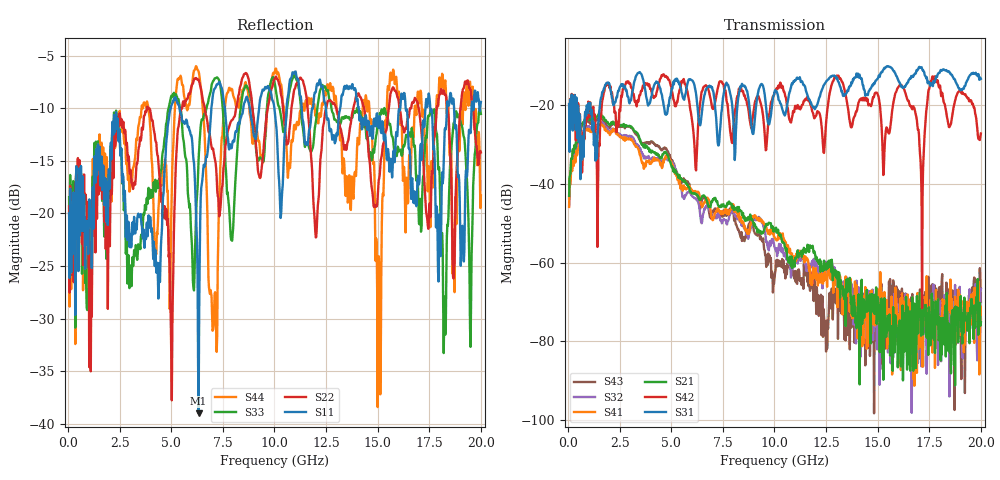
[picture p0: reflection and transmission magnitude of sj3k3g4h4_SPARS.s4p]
! FILE: E:\users\goganessyan\GBX_Backplane\FR408_backplane\1m_INBOUND_FEXT\sj3k3g4h4_SPARS.s4p
# MHZ S RI R 50.00
! FREQ  S11  S12  S13  S14
!  S21  S22  S23  S24
!  S31  S32  S33  S34
!  S41  S42  S43  S44
!  REAL  IMAG  REAL  IMAG  REAL  IMAG  REAL  IMAG
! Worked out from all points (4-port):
!   799 points, 50 MHz to 20 GHz, reference 50 ohm
!   strongest paths, dB at 50 MHz, 5.025 GHz, 10.03 GHz, 15.03 GHz, 20 GHz:
!     S31: -19.7, -15.8, -16.2, -13.1, -13.3
!     S42: -19.7, -16.3, -16.7, -17.6, -27.2
!     S21: -43.0, -35.7, -51.9, -69.0, -75.2
!     S41: -45.8, -35.0, -53.8, -71.5, -74.2
!     S32: -45.4, -34.4, -56.3, -77.7, -66.7
!     S43: -43.7, -34.3, -62.7, -74.3, -70.0
!   lowest |S11| = -39.0 dB at 6.325 GHz (marker M1), VSWR 1.02, Z = 49 + j0.376 ohm
!   |S11| at or under -10 dB: start of sweep to 4.979 GHz; 5.397 GHz to 6.944 GHz (1.546 GHz wide, 25.1 % of centre); 14.08 GHz to 16.09 GHz (2.012 GHz wide, 13.3 % of centre)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
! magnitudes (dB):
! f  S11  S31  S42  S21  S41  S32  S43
! 50 MHz  -20.0  -19.7  -19.7  -43.0  -45.8  -45.4  -43.7
! 5.025 GHz  -9.7  -15.8  -16.3  -35.7  -35.0  -34.4  -34.3
! 6.325 GHz  -39.0  -23.6  -23.4  -43.4  -42.2  -45.0  -44.4
! 7.15 GHz  -8.0  -21.9  -18.5  -43.8  -47.2  -48.4  -46.3
! 12.47 GHz  -9.7  -14.3  -26.3  -61.5  -63.8  -59.8  -76.5
! 18.25 GHz  -12.0  -11.1  -19.8  -76.6  -69.6  -68.2  -69.2
! 20 GHz  -9.4  -13.3  -27.2  -75.2  -74.2  -66.7  -70.0
